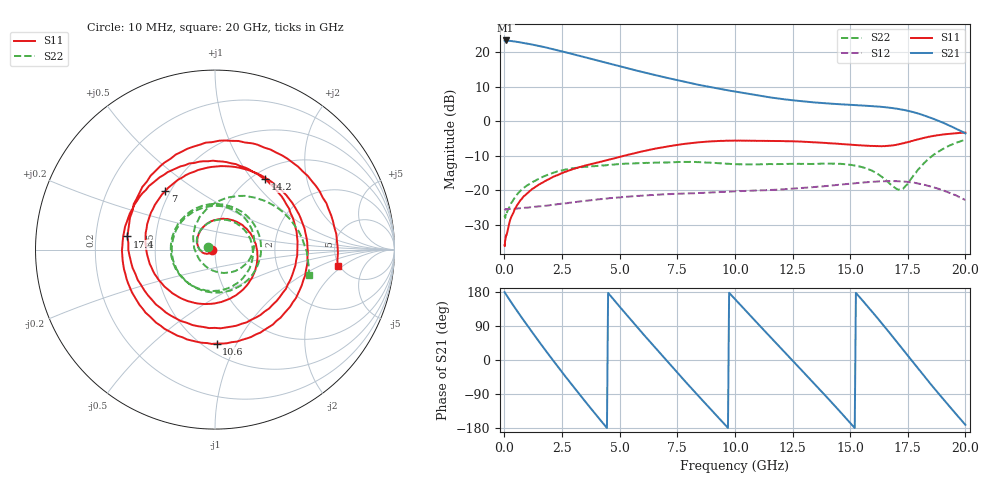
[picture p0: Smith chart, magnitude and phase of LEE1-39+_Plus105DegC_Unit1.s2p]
!Keysight Technologies,N5245A,MY52442000,A.10.65.23
!Date: Tuesday, November 25, 2025 21:58:43
!Correction: S11(Full 2 Port(1,2))
!S21(Full 2 Port(1,2))
!S12(Full 2 Port(1,2))
!S22(Full 2 Port(1,2))
!S2P File: Measurements: S11, S21, S12, S22:
!Deduct Board Loss
# Hz S  dB  R 50
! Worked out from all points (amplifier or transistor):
!   408 points, 10 MHz to 20 GHz, reference 50 ohm
!   highest |S21| = 23.5 dB at 50 MHz (marker M1)
!   |S21| within 3 dB of that: start of sweep to 2.41 GHz
!   unconditionally stable (mu >= 1): start of sweep to end of sweep
!   at 3.05 GHz: K = 1.04, MAG = 20.1 dB, |S12| = -23.4 dB
!   at 9.85 GHz: K = 1.44, MAG = 10.6 dB, |S12| = -20.3 dB
!   at 20 GHz: K = 3.94, MAG = 0.8 dB, |S12| = -22.8 dB
!   S11 on the Smith chart (normalised r, x): 10 MHz: 0.97, -0.00; 7 GHz: 0.47, +0.37; 10.6 GHz: 0.58, -0.83; 14.2 GHz: 1.14, +1.17; 17.4 GHz: 0.34, +0.07; 20 GHz: 4.81, -1.71
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1e7  -35.89 -172.6  23.36 179.1  -25.40 0.1  -27.63 159.2
5e7  -33.97 -162.0  23.45 175.2  -25.57 -2.4  -27.13 -173.9
5e8  -24.93 -157.6  23.10 133.9  -25.29 -23.7  -21.60 -178.5
9e8  -21.43 -179.9  22.65 99.2  -25.02 -44.1  -18.97 154.8
1.3e9  -19.25 154.5  22.14 65.5  -24.76 -64.3  -17.31 125.2
1.85e9  -16.98 118.1  21.35 20.1  -24.38 -93.1  -15.57 84.4
2.65e9  -14.62 65.0  20.04 -43.7  -23.74 -135.5  -13.96 27.3
3.35e9  -13.08 17.7  18.82 -97.6  -23.14 -174.0  -13.25 -21.7
4.25e9  -11.57 -44.6  17.26 -164.8  -22.46 135.3  -12.76 -85.2
5.25e9  -9.87 -114.5  15.53 122.9  -21.88 77.8  -12.24 -154.7
5.9e9  -8.81 -158.0  14.45 77.1  -21.53 39.9  -12.10 161.8
6.7e9  -7.70 150.0  13.18 21.4  -21.23 -6.9  -11.92 109.4
7e9  -7.38 130.5  12.71 0.9  -21.12 -24.3  -11.90 89.9
8.3e9  -6.15 49.2  10.76 -86.9  -20.80 -100.3  -11.75 9.4
1.005e10  -5.59 -55.0  8.59 157.7  -20.24 158.2  -12.43 -89.3
1.06e10  -5.62 -88.9  7.96 121.7  -20.13 126.6  -12.47 -119.4
1.21e10  -5.71 -179.5  6.44 24.4  -19.70 39.4  -12.34 164.7
1.335e10  -6.00 106.5  5.55 -56.5  -19.08 -33.4  -12.33 108.3
1.42e10  -6.35 54.4  5.12 -112.0  -18.56 -83.8  -12.25 69.9
1.67e10  -7.04 -128.1  3.97 72.5  -17.29 115.5  -17.95 -82.5
1.74e10  -6.13 171.4  3.22 19.2  -17.49 66.4  -18.71 176.6
2e10  -3.23 -7.8  -3.49 -171.1  -22.80 -108.2  -5.32 -15.4
